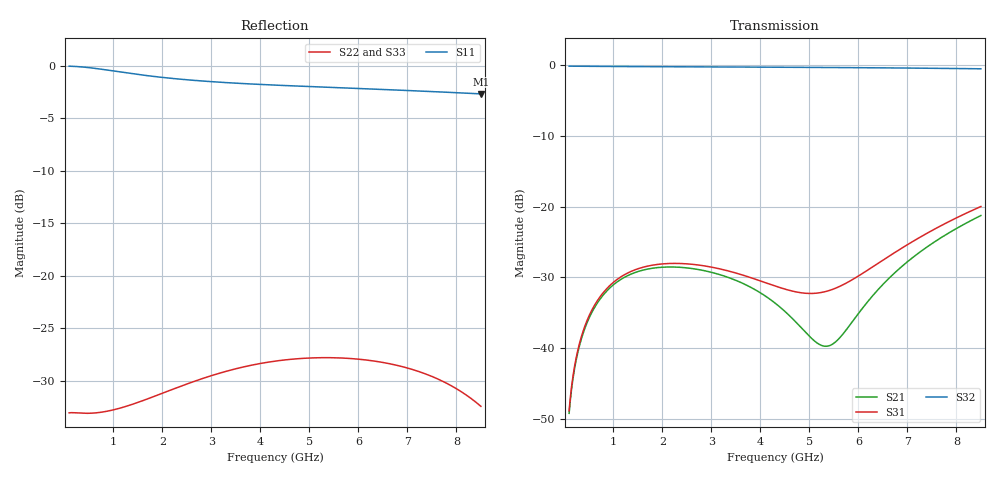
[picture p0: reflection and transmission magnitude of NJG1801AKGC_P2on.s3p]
! Port1:P1, Port2:P2, Port3:PC, VCTL1=3V, VCTL2=0V
# hz S ma R 50
! 3 Port Network Data from SP1.SP block
! freq  magS11  angS11  magS12  angS12  magS13  angS13
!  magS21  angS21
!  magS22  angS22  magS23  angS23
!  magS31  angS31  magS32  angS32
!  magS33  angS33
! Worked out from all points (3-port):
!   841 points, 100 MHz to 8.5 GHz, reference 50 ohm
!   strongest paths, dB at 100 MHz, 2.2 GHz, 4.3 GHz, 6.4 GHz, 8.5 GHz:
!     S32: -0.2, -0.3, -0.4, -0.5, -0.6
!     S31: -48.8, -28.0, -31.2, -28.0, -20.0
!     S21: -49.1, -28.5, -33.6, -31.7, -21.3
!   lowest |S11| = -2.7 dB at 8.5 GHz (marker M1), VSWR 6.52, Z = 14.6 + j46.4 ohm
!   |S11| at or under -10 dB: nowhere
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1e8  0.9944 -7.4  0.003493 74.5  0.003639 74.6
     0.003495 74.4  0.0223 -2.6  0.9737 -1.2
     0.003641 74.5  0.9737 -1.2  0.02241 -1.9
2.7e8  0.9899 -19.8  0.009126 73.9  0.009474 74.6
       0.009128 73.8  0.02227 -8.8  0.9728 -3.0
       0.009477 74.5  0.9728 -3.0  0.02245 -8.8
5.2e8  0.9777 -37.6  0.01673 65.5  0.01735 66.6
       0.01673 65.5  0.0222 -17.5  0.9713 -5.8
       0.01736 66.6  0.9713 -5.8  0.02227 -18.5
9.4e8  0.9491 -64.8  0.02689 50.8  0.02796 52.6
       0.0269 50.8  0.02286 -31.7  0.9691 -10.3
       0.02797 52.6  0.9691 -10.3  0.02297 -33.8
1.36e9  0.9181 -88.5  0.03336 37.5  0.03484 40.3
        0.03337 37.5  0.02435 -44.5  0.9674 -14.9
        0.03485 40.3  0.9674 -14.9  0.02456 -47.4
2.62e9  0.8522 -140.2  0.03651 8.6  0.03913 15.7
        0.03652 8.6  0.03129 -74.0  0.9634 -28.5
        0.03914 15.7  0.9634 -28.5  0.03169 -79.2
4.3e9  0.8081 174.9  0.02089 -7.1  0.02756 12.7
       0.0209 -7.1  0.03928 -100.9  0.9575 -47.0
       0.02757 12.7  0.9575 -47.0  0.04004 -109.1
5.43e9  0.7882 150.9  0.01053 46.7  0.02576 42.8
        0.01053 46.6  0.0408 -114.2  0.9529 -59.6
        0.02577 42.8  0.9529 -59.6  0.04172 -125.4
6.9e9  0.7635 122.2  0.03814 90.2  0.05125 65.0
       0.03814 90.2  0.03697 -127.7  0.9453 -76.4
       0.05125 65.0  0.9453 -76.4  0.03778 -143.9
8.5e9  0.7342 91.6  0.08637 76.9  0.09997 56.1
       0.08638 76.9  0.02395 -134.0  0.933 -95.4
       0.09998 56.1  0.933 -95.4  0.02394 -160.7
